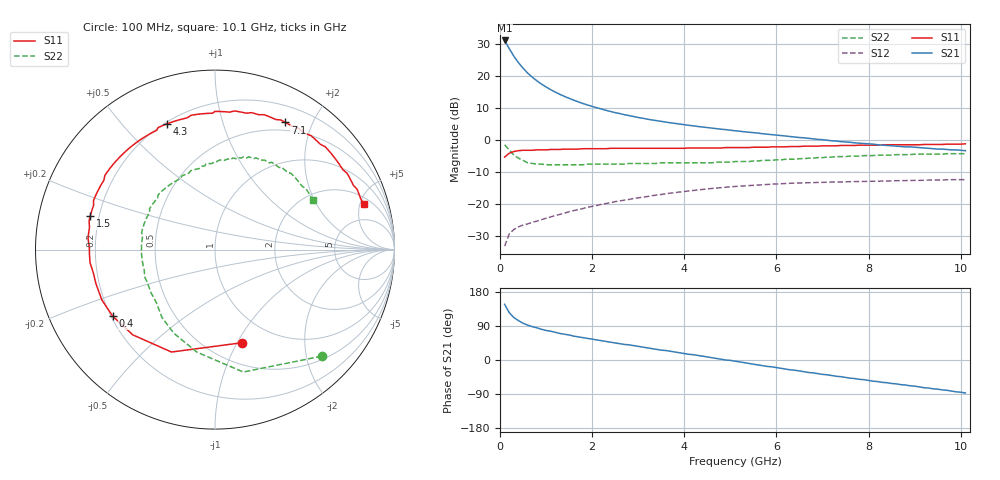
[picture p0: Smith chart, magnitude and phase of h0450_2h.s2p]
!HBFP-0450
!S and NOISE PARAMETERS at Vce=2V  Ic=50mA.  LAST UPDATED  09-04-98
# GHZ S MA R  50
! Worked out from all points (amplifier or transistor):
!   101 points, 100 MHz to 10.1 GHz, reference 50 ohm
!   highest |S21| = 31.1 dB at 100 MHz (marker M1)
!   |S21| within 3 dB of that: start of sweep to 219.3 MHz
!   unconditionally stable (mu >= 1): 2.071 GHz to end of sweep
!   at 1.7 GHz: K = 0.96, MSG = 16.8 dB, |S12| = -21.7 dB
!   at 5.1 GHz: K = 1.08, MAG = 6.9 dB, |S12| = -14.5 dB
!   at 10.1 GHz: K = 1.04, MAG = 3.2 dB, |S12| = -12.4 dB
!   lowest NFmin = 1.78 dB at 1.8 GHz
!   S11 on the Smith chart (normalised r, x): 100 MHz: 0.71, -1.04; 400 MHz: 0.21, -0.28; 1.5 GHz: 0.17, +0.13; 4.3 GHz: 0.21, +0.67; 7.1 GHz: 0.39, +1.63; 10.1 GHz: 2.62, +5.47
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0.1  0.54 -74.0  35.69 147.0  0.022 63.0  0.84 -45.0
0.2  0.62 -113.0  26.62 125.0  0.034 48.0  0.7 -77.0
0.3  0.66 -134.0  20.32 112.0  0.04 41.0  0.58 -100.0
0.4  0.68 -147.0  16.08 104.0  0.044 37.0  0.52 -116.0
0.5  0.69 -156.0  13.2 97.0  0.047 36.0  0.48 -128.0
0.6  0.69 -164.0  11.06 92.0  0.049 36.0  0.44 -138.0
0.7  0.69 -169.0  9.54 88.0  0.052 36.0  0.43 -146.0
0.8  0.7 -174.0  8.37 85.0  0.054 37.0  0.42 -153.0
0.9  0.7 -178.0  7.45 81.0  0.057 37.0  0.42 -159.0
1.1  0.71 175.0  6.09 76.0  0.063 38.0  0.41 -168.0
1.3  0.71 170.0  5.15 70.0  0.069 38.0  0.41 -176.0
1.5  0.72 165.0  4.46 66.0  0.076 38.0  0.41 178.0
1.8  0.73 158.0  3.7 59.0  0.085 37.0  0.41 169.0
2.1  0.73 151.0  3.18 53.0  0.095 35.0  0.42 162.0
2.5  0.74 144.0  2.67 45.0  0.109 32.0  0.42 154.0
3.5  0.74 125.0  1.95 26.0  0.141 22.0  0.44 136.0
4.3  0.75 111.0  1.62 12.0  0.166 12.0  0.44 122.0
5.1  0.76 97.0  1.39 -3.0  0.188 1.0  0.46 107.0
6.8  0.8 66.0  1.04 -34.0  0.216 -24.0  0.52 77.0
7.1  0.81 61.0  0.99 -39.0  0.219 -28.0  0.54 73.0
8.5  0.84 40.0  0.81 -62.0  0.23 -47.0  0.58 52.0
10.1  0.87 17.0  0.68 -87.0  0.24 -70.0  0.61 27.0
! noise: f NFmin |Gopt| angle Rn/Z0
1.8  1.78  0.6  -153  0.09
2  1.81  0.59  -151  0.11
2.5  1.94  0.62  -141  0.16
3.5  2.19  0.65  -124  0.33
4  2.31  0.68  -114  0.48
5  2.57  0.71  -96  0.85
5.5  2.69  0.73  -86  1.18
7  3.07  0.77  -60  2.36
8  3.32  0.8  -44  3.43
10  3.83  0.82  -16  5.48
